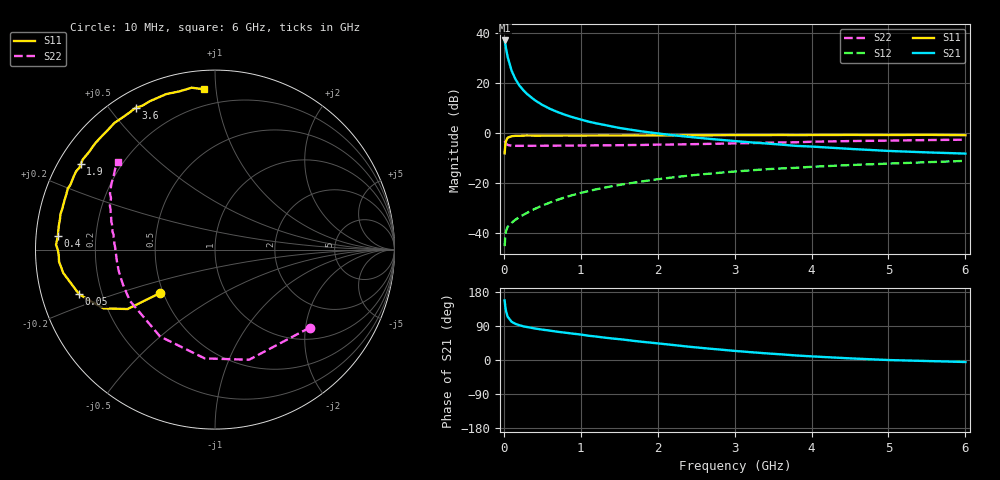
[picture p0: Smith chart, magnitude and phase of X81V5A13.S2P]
! SIEMENS Small Signal Semiconductors
! BFP136W
! Si NPN RF Bipolar Junction Transistor in SOT343
! VCE = 1.5 V  IC = 130 mA
! Common Emitter S-Parameters:  September  1994
# GHz  S  MA  R  50
!  f  S11  S21  S12  S22
! GHz  MAG  ANG  MAG  ANG  MAG  ANG  MAG  ANG
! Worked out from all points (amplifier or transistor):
!   40 points, 10 MHz to 6 GHz, reference 50 ohm
!   highest |S21| = 37.0 dB at 10 MHz (marker M1)
!   |S21| within 3 dB of that: start of sweep to 27.5 MHz
!   unconditionally stable (mu >= 1): 393.6 MHz to 3.405 GHz; 3.709 GHz to 3.913 GHz; 5.873 GHz to end of sweep
!   at 200 MHz: K = 0.79, MSG = 26.4 dB, |S12| = -33.7 dB
!   at 1.5 GHz: K = 1.13, MAG = 9.2 dB, |S12| = -20.8 dB
!   at 6 GHz: K = 1.01, MAG = 0.7 dB, |S12| = -11.2 dB
!   S11 on the Smith chart (normalised r, x): 10 MHz: 0.48, -0.27; 50 MHz: 0.12, -0.16; 400 MHz: 0.06, +0.04; 1.9 GHz: 0.06, +0.29; 3.6 GHz: 0.07, +0.58; 6 GHz: 0.10, +0.93
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0.01  0.3885 -141.6  70.42 157.3  0.0054 64.6  0.684 -39.4
0.02  0.5888 -145.8  58.31 139.3  0.0089 51.7  0.6424 -72.8
0.03  0.7026 -152.2  47.32 127.5  0.0111 45.5  0.6089 -95.4
0.05  0.797 -161.8  32.66 114.2  0.0132 37.3  0.5727 -122.3
0.1  0.8557 -171.3  17.64 101.1  0.0158 37.5  0.5535 -149.0
0.15  0.8715 -175.6  11.92 95.4  0.0182 41.6  0.5485 -159.2
0.2  0.8712 -178.1  8.931 91.8  0.0206 45.0  0.5484 -164.7
0.25  0.8768 179.8  7.205 89.0  0.0227 48.4  0.5495 -168.1
0.3  0.8863 178.3  6.019 87.1  0.025 51.5  0.5491 -170.5
0.4  0.8787 175.1  4.529 83.3  0.03 55.3  0.5506 -173.7
0.5  0.8795 172.8  3.613 80.1  0.0351 58.4  0.5514 -175.9
0.7  0.8803 168.7  2.601 74.4  0.0458 62.0  0.5538 -178.6
0.9  0.8806 165.2  2.038 69.5  0.0571 62.8  0.5559 179.0
1.1  0.8827 161.0  1.676 64.0  0.0682 62.9  0.5595 177.3
1.5  0.884 154.5  1.255 55.0  0.0907 61.5  0.5655 174.1
1.9  0.8871 147.5  1.018 46.0  0.1123 58.4  0.5755 170.9
2.2  0.888 142.3  0.895 39.6  0.1285 55.6  0.583 168.3
3.2  0.8989 125.2  0.646 20.8  0.177 45.4  0.6225 159.1
3.6  0.9055 119.2  0.582 15.0  0.1935 41.3  0.6404 155.5
4.5  0.908 107.4  0.477 4.3  0.2264 32.6  0.6843 147.5
5.5  0.9114 98.2  0.406 -2.7  0.2583 24.5  0.7163 140.9
6  0.8951 94.0  0.384 -5.3  0.2746 20.0  0.7282 137.9
